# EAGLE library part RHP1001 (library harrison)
Intan Technologies RHP1001 patch clamp chip (QFN-48 package)
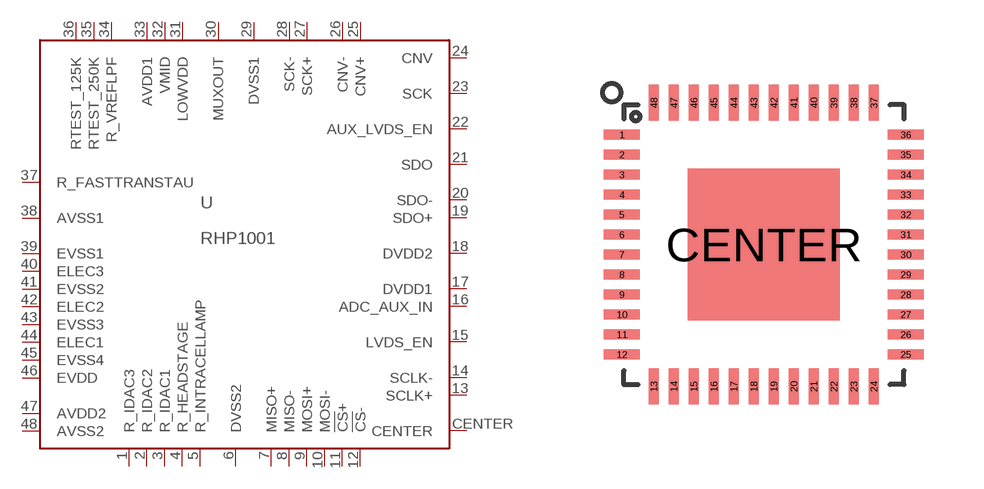
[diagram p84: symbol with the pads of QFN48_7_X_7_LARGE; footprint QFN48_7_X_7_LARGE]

Designator prefix U

## RHP1001_QFN  [QFN48_7_X_7_LARGE]
1  R_IDAC3  pas
2  R_IDAC2  pas
3  R_IDAC1  pas
4  R_HEADSTAGE  pas
5  R_INTRACELLAMP  pas
6  DVSS2  pwr
7  MISO+  out
8  MISO-  out
9  MOSI+  in
10  MOSI-  in
11  !CS!+  in
12  !CS!-  in
13  SCLK+  in
14  SCLK-  in
15  LVDS_EN  in
16  ADC_AUX_IN  in
17  DVDD1  pwr
18  DVDD2  pwr
19  SDO+  out
20  SDO-  out
21  SDO  in
22  AUX_LVDS_EN  in
23  SCK  out
24  CNV  out
25  CNV+  in
26  CNV-  in
27  SCK+  in
28  SCK-  in
29  DVSS1  pwr
30  MUXOUT  out
31  LOWVDD  pwr
32  VMID  pwr
33  AVDD1  pwr
34  R_VREFLPF  pas
35  RTEST_250K  pas
36  RTEST_125K  pas
37  R_FASTTRANSTAU  pas
38  AVSS1  pwr
39  EVSS1  pwr
40  ELEC3  in
41  EVSS2  pwr
42  ELEC2  in
43  EVSS3  pwr
44  ELEC1  in
45  EVSS4  pwr
46  EVDD  pwr
47  AVDD2  pwr
48  AVSS2  pwr
CENTER  CENTER  pwr

## Footprint QFN48_7_X_7_LARGE (pad centres in mm)
smd 0.9 x 0.25: 1 -3.55,2.75; 2 -3.55,2.25; 3 -3.55,1.75; 4 -3.55,1.25; 5 -3.55,0.75; 6 -3.55,0.25; 7 -3.55,-0.25; 8 -3.55,-0.75; 9 -3.55,-1.25; 10 -3.55,-1.75; 11 -3.55,-2.25; 12 -3.55,-2.75; 25 3.55,-2.75; 26 3.55,-2.25; 27 3.55,-1.75; 28 3.55,-1.25; 29 3.55,-0.75; 30 3.55,-0.25; 31 3.55,0.25; 32 3.55,0.75; 33 3.55,1.25; 34 3.55,1.75; 35 3.55,2.25; 36 3.55,2.75
smd 0.25 x 0.9: 13 -2.75,-3.55; 14 -2.25,-3.55; 15 -1.75,-3.55; 16 -1.25,-3.55; 17 -0.75,-3.55; 18 -0.25,-3.55; 19 0.25,-3.55; 20 0.75,-3.55; 21 1.25,-3.55; 22 1.75,-3.55; 23 2.25,-3.55; 24 2.75,-3.55; 37 2.75,3.55; 38 2.25,3.55; 39 1.75,3.55; 40 1.25,3.55; 41 0.75,3.55; 42 0.25,3.55; 43 -0.25,3.55; 44 -0.75,3.55; 45 -1.25,3.55; 46 -1.75,3.55; 47 -2.25,3.55; 48 -2.75,3.55
smd 3.8 x 3.8: CENTER 0,0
